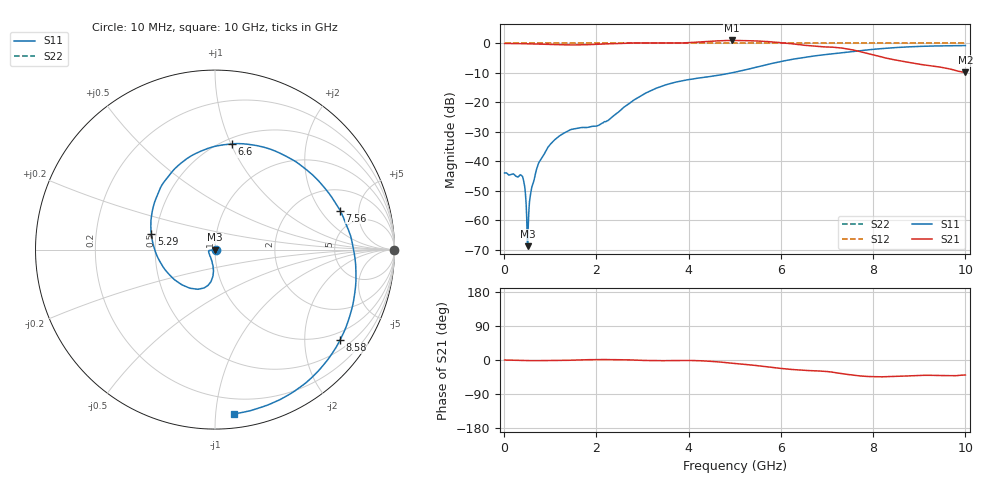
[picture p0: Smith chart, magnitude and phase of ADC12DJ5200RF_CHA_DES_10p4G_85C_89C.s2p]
! Texas Instruments, Inc.
! ADC12DJ5200RF - CH A S-Parameters (DES Mode, Fs = 10.4 GSPS, 85 degC case, 89 degC juntion)
! Port 1 represents the 100-ohm differenal input, Port 2 the digital output
! freq  dbS11  angS11  dbS21 angS21 dbS12 angS12 dbS22 angS22
# HZ S DB R 100
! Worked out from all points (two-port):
!   1000 points, 10 MHz to 10 GHz, reference 100 ohm
!   highest |S21| = 1.02 dB at 4.93 GHz (marker M1); lowest = -9.8 dB at 10 GHz (marker M2)
!   |S21| within 3 dB of the highest: start of sweep to 7.486 GHz
!   lowest |S11| = -68.9 dB at 510 MHz (marker M3), VSWR 1.00, Z = 100 - j0.0713 ohm
!   |S11| at or under -10 dB: start of sweep to 4.932 GHz
!   |S22| runs from 0.0 to 0.0 dB; largest |S21 - S12| = 0.78
!   S11 on the Smith chart (normalised r, x): 10 MHz: 1.01, -0.00; 5.29 GHz: 0.47, +0.10; 6.6 GHz: 0.55, +1.01; 7.56 GHz: 3.35, +3.13; 8.58 GHz: 0.75, -2.91; 10 GHz: 0.09, -1.12
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1e7  -43.98 -7.6  0.00 -0.0  0.00 0.0  0.00 0.0
3.8e8  -44.92 -10.5  -0.05 -1.3  0.00 0.0  0.00 0.0
4.3e8  -47.24 -0.5  -0.08 -1.4  0.00 0.0  0.00 0.0
4.7e8  -52.81 6.8  -0.09 -1.5  0.00 0.0  0.00 0.0
5.1e8  -68.87 -81.6  -0.11 -1.6  0.00 0.0  0.00 0.0
7.1e8  -42.37 -157.4  -0.21 -1.7  0.00 0.0  0.00 0.0
9.4e8  -35.52 -169.1  -0.30 -1.7  0.00 0.0  0.00 0.0
1.26e9  -30.80 -171.7  -0.44 -1.1  0.00 0.0  0.00 0.0
1.68e9  -28.56 -163.4  -0.46 0.4  0.00 0.0  0.00 0.0
2.24e9  -26.25 -119.8  -0.12 1.0  0.00 0.0  0.00 0.0
3.34e9  -14.98 -96.9  0.13 -1.8  0.00 0.0  0.00 0.0
4.2e9  -11.79 -123.9  0.48 -1.7  0.00 0.0  0.00 0.0
4.93e9  -10.01 -168.8  1.02 -8.4  0.00 0.0  0.00 0.0
5.01e9  -9.74 -174.4  1.02 -9.3  0.00 0.0  0.00 0.0
5.29e9  -8.74 165.9  0.92 -12.5  0.00 0.0  0.00 0.0
5.9e9  -6.49 126.2  0.42 -20.8  0.00 0.0  0.00 0.0
6.6e9  -4.49 81.1  -0.73 -27.9  0.00 0.0  0.00 0.0
6.67e9  -4.33 76.5  -0.85 -28.3  0.00 0.0  0.00 0.0
7.56e9  -2.73 17.4  -2.19 -40.1  0.00 0.0  0.00 0.0
8.34e9  -1.56 -25.8  -5.17 -43.7  0.00 0.0  0.00 0.0
8.58e9  -1.31 -35.9  -5.89 -42.7  0.00 0.0  0.00 0.0
1e10  -0.71 -83.2  -9.84 -39.6  0.00 0.0  0.00 0.0
